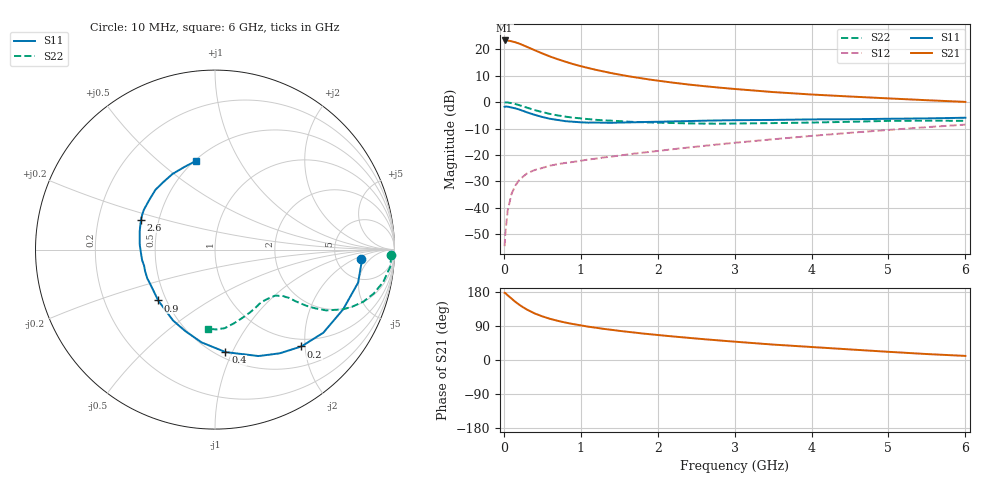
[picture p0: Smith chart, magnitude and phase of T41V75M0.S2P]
! Infineon Technologies  Discrete & RF Semiconductors
! BFR182T
! Si NPN RF Bipolar Junction Transistor in SC75
! VCE = 1.75 V  IC = 5 mA
! Common Emitter S-Parameters:  October  1999
# GHz  S  MA  R  50
!  f  S11  S21  S12  S22
! GHz  MAG  ANG  MAG  ANG  MAG  ANG  MAG  ANG
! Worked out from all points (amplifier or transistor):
!   36 points, 10 MHz to 6 GHz, reference 50 ohm
!   highest |S21| = 23.3 dB at 10 MHz (marker M1)
!   |S21| within 3 dB of that: start of sweep to 347 MHz
!   unconditionally stable (mu >= 1): 1.348 GHz to 4.049 GHz
!   at 250 MHz: K = 0.29, MSG = 24.8 dB, |S12| = -28.2 dB
!   at 1.4 GHz: K = 1.02, MAG = 14.9 dB, |S12| = -20.6 dB
!   at 6 GHz: K = 0.85, MSG = 4.3 dB, |S12| = -8.5 dB
!   lowest NFmin = 1.20 dB at 450 MHz
!   S11 on the Smith chart (normalised r, x): 10 MHz: 8.86, -2.75; 200 MHz: 0.85, -1.92; 400 MHz: 0.55, -0.94; 900 MHz: 0.45, -0.31; 2.6 GHz: 0.40, +0.17; 6 GHz: 0.51, +0.67
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0.01  0.8136 -3.7  14.55 177.4  0.0019 84.5  0.9819 -1.9
0.02  0.8213 -3.9  14.51 176.6  0.0034 96.2  0.9826 -2.2
0.05  0.8183 -13.0  14.5 170.7  0.0089 84.0  0.981 -5.6
0.1  0.7877 -25.0  14.04 162.1  0.0185 79.4  0.9552 -10.8
0.15  0.7608 -37.5  13.43 153.4  0.0265 72.0  0.9174 -15.5
0.2  0.7229 -48.3  12.7 145.9  0.0337 68.6  0.8752 -19.4
0.25  0.6809 -58.1  11.84 139.2  0.039 62.9  0.8279 -22.6
0.3  0.6405 -67.8  11.03 133.1  0.0448 60.4  0.7854 -25.1
0.4  0.5738 -84.2  9.536 122.9  0.052 54.8  0.7055 -28.7
0.5  0.5224 -98.2  8.28 115.2  0.057 52.8  0.6456 -30.4
0.6  0.4831 -110.1  7.247 108.7  0.0629 51.7  0.5971 -31.6
0.7  0.459 -120.6  6.443 103.4  0.0671 51.5  0.5596 -32.2
0.9  0.425 -138.2  5.212 94.9  0.0739 51.7  0.5068 -32.9
1.1  0.4087 -152.0  4.379 87.9  0.0822 52.7  0.4757 -33.8
1.3  0.4075 -163.2  3.772 82.1  0.0901 54.0  0.4515 -34.8
1.6  0.412 -176.1  3.108 74.6  0.1018 56.0  0.4274 -36.8
2.2  0.4313 166.7  2.323 62.1  0.1288 59.4  0.402 -43.0
2.6  0.4448 157.9  1.998 54.9  0.1488 60.5  0.3922 -48.1
3.5  0.4598 142.2  1.544 40.7  0.1982 60.8  0.4004 -60.5
4.5  0.4736 127.5  1.272 27.9  0.2626 58.1  0.4239 -75.5
5.5  0.4912 110.2  1.083 15.7  0.3358 53.3  0.4449 -89.0
6  0.5056 102.0  1.007 10.8  0.3748 49.8  0.4427 -94.9
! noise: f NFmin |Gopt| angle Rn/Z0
0.45  1.2  0.27  37  0.3
0.9  1.3  0.25  75  0.23
1.8  1.9  0.21  145  0.2
